FUNCTION "PR_GestioSalvastampi_WW" : VOID
TITLE =Gestione Salvastampi Cliente*
AUTHOR : 'A.A.E'
FAMILY : SALVASTA
NAME : SALVASTA
VERSION : 0.1


VAR_TEMP
  ST_CTRL : BOOL ;	//START CONTROLLO
  Camma_PMS : BOOL ;	//Appoggio per camma a pms
  CTRL_Syncr : BOOL ;	//Controllo Sincronismo
  Ang_Fren : INT ;	//Angolo Frenatura a PMS
  CMD_Prg : BOOL ;	//Comando Programmazione Camma
  Antic_Dyn : INT ;	//Gradi Anticipo Camme Dinamiche
  Page_Ok : BOOL ;	//Pagina Visualizzata HMI Corretta
  Results : INT ;
  ByPass_Cntr : BOOL ;
END_VAR
BEGIN
NETWORK
TITLE =R/Reset allarmi salvastampo*
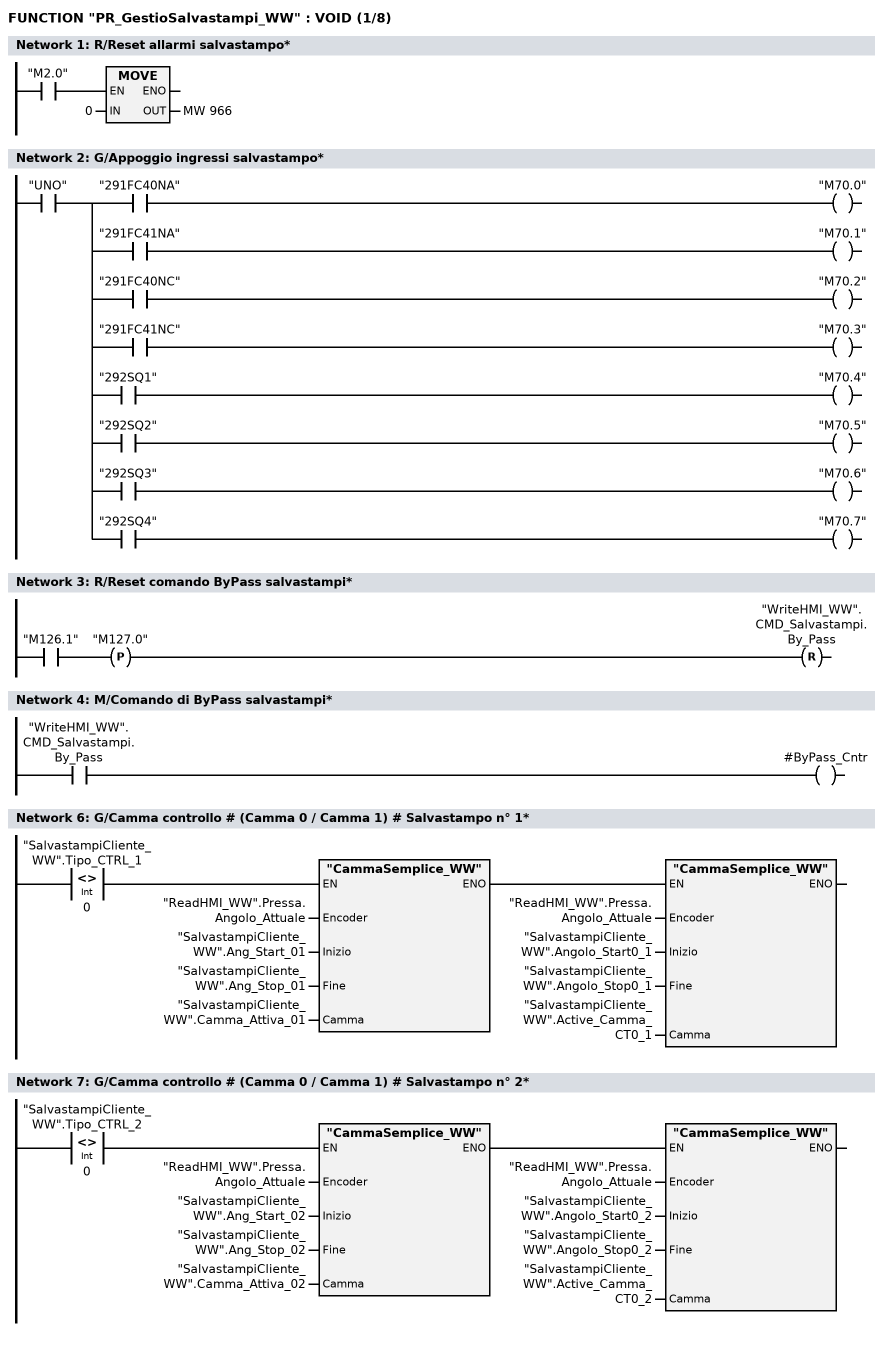
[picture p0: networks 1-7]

      U     "M2.0";
      SPBNB _001;
      L     0;
      T     MW   966;
_001: NOP   0;
NETWORK
TITLE =G/Appoggio ingressi salvastampo*

      U     "UNO";
      =     L     13.0;
      U     L     13.0;
      U     "291FC40NA";
      =     "M70.0";
      U     L     13.0;
      U     "291FC41NA";
      =     "M70.1";
      U     L     13.0;
      U     "291FC40NC";
      =     "M70.2";
      U     L     13.0;
      U     "291FC41NC";
      =     "M70.3";
      U     L     13.0;
      U     "292SQ1";
      =     "M70.4";
      U     L     13.0;
      U     "292SQ2";
      =     "M70.5";
      U     L     13.0;
      U     "292SQ3";
      =     "M70.6";
      U     L     13.0;
      U     "292SQ4";
      =     "M70.7";
NETWORK
TITLE =R/Reset comando ByPass salvastampi*

      U     "M126.1";
      FP    "M127.0";
      R     "WriteHMI_WW".CMD_Salvastampi.By_Pass;
NETWORK
TITLE =M/Comando di ByPass salvastampi*

      U     "WriteHMI_WW".CMD_Salvastampi.By_Pass;
      =     #ByPass_Cntr;
NETWORK
TITLE =######################## CAMME SALVASTAMPO #####################



NETWORK
TITLE =G/Camma controllo # (Camma 0 / Camma 1) # Salvastampo n° 1*

      U(    ;
      U(    ;
      L     "SalvastampiCliente_WW".Tipo_CTRL_1;
      L     0;
      <>I   ;
      )     ;
      SPBNB _002;
      CALL "CammaSemplice_WW" (
           Encoder                  := "ReadHMI_WW".Pressa.Angolo_Attuale,
           Inizio                   := "SalvastampiCliente_WW".Ang_Start_01,
           Fine                     := "SalvastampiCliente_WW".Ang_Stop_01,
           Camma                    := "SalvastampiCliente_WW".Camma_Attiva_01);
_002: U     BIE;
      )     ;
      SPBNB _003;
      CALL "CammaSemplice_WW" (
           Encoder                  := "ReadHMI_WW".Pressa.Angolo_Attuale,
           Inizio                   := "SalvastampiCliente_WW".Angolo_Start0_1,
           Fine                     := "SalvastampiCliente_WW".Angolo_Stop0_1,
           Camma                    := "SalvastampiCliente_WW".Active_Camma_CT0_1);
_003: NOP   0;
NETWORK
TITLE =G/Camma controllo # (Camma 0 / Camma 1) # Salvastampo n° 2*

      U(    ;
      U(    ;
      L     "SalvastampiCliente_WW".Tipo_CTRL_2;
      L     0;
      <>I   ;
      )     ;
      SPBNB _004;
      CALL "CammaSemplice_WW" (
           Encoder                  := "ReadHMI_WW".Pressa.Angolo_Attuale,
           Inizio                   := "SalvastampiCliente_WW".Ang_Start_02,
           Fine                     := "SalvastampiCliente_WW".Ang_Stop_02,
           Camma                    := "SalvastampiCliente_WW".Camma_Attiva_02);
_004: U     BIE;
      )     ;
      SPBNB _005;
      CALL "CammaSemplice_WW" (
           Encoder                  := "ReadHMI_WW".Pressa.Angolo_Attuale,
           Inizio                   := "SalvastampiCliente_WW".Angolo_Start0_2,
           Fine                     := "SalvastampiCliente_WW".Angolo_Stop0_2,
           Camma                    := "SalvastampiCliente_WW".Active_Camma_CT0_2);
_005: NOP   0;
NETWORK
TITLE =G/Camma controllo # (Camma 0 / Camma 1) # Salvastampo n° 3*
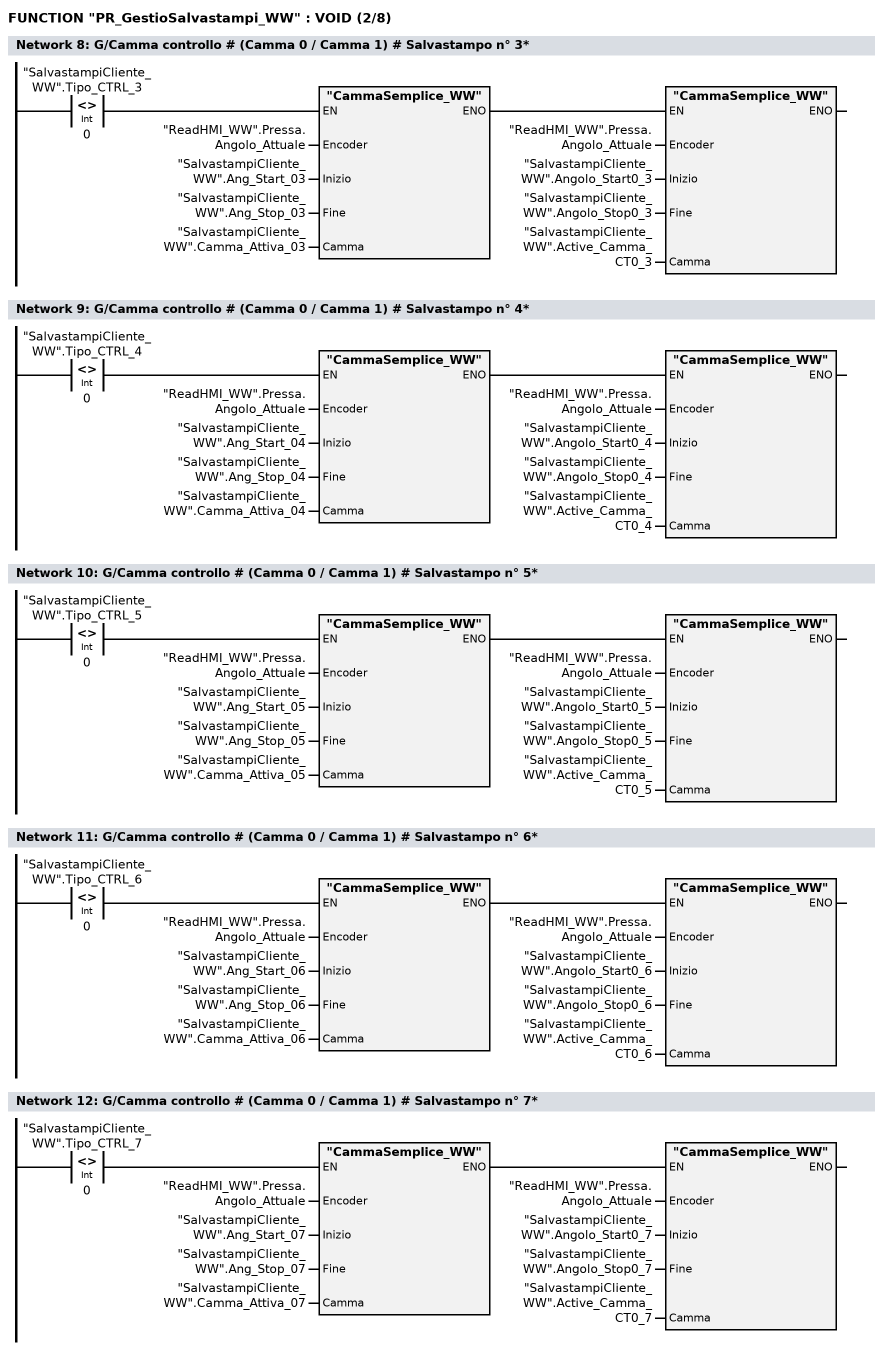
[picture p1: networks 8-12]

      U(    ;
      U(    ;
      L     "SalvastampiCliente_WW".Tipo_CTRL_3;
      L     0;
      <>I   ;
      )     ;
      SPBNB _006;
      CALL "CammaSemplice_WW" (
           Encoder                  := "ReadHMI_WW".Pressa.Angolo_Attuale,
           Inizio                   := "SalvastampiCliente_WW".Ang_Start_03,
           Fine                     := "SalvastampiCliente_WW".Ang_Stop_03,
           Camma                    := "SalvastampiCliente_WW".Camma_Attiva_03);
_006: U     BIE;
      )     ;
      SPBNB _007;
      CALL "CammaSemplice_WW" (
           Encoder                  := "ReadHMI_WW".Pressa.Angolo_Attuale,
           Inizio                   := "SalvastampiCliente_WW".Angolo_Start0_3,
           Fine                     := "SalvastampiCliente_WW".Angolo_Stop0_3,
           Camma                    := "SalvastampiCliente_WW".Active_Camma_CT0_3);
_007: NOP   0;
NETWORK
TITLE =G/Camma controllo # (Camma 0 / Camma 1) # Salvastampo n° 4*

      U(    ;
      U(    ;
      L     "SalvastampiCliente_WW".Tipo_CTRL_4;
      L     0;
      <>I   ;
      )     ;
      SPBNB _008;
      CALL "CammaSemplice_WW" (
           Encoder                  := "ReadHMI_WW".Pressa.Angolo_Attuale,
           Inizio                   := "SalvastampiCliente_WW".Ang_Start_04,
           Fine                     := "SalvastampiCliente_WW".Ang_Stop_04,
           Camma                    := "SalvastampiCliente_WW".Camma_Attiva_04);
_008: U     BIE;
      )     ;
      SPBNB _009;
      CALL "CammaSemplice_WW" (
           Encoder                  := "ReadHMI_WW".Pressa.Angolo_Attuale,
           Inizio                   := "SalvastampiCliente_WW".Angolo_Start0_4,
           Fine                     := "SalvastampiCliente_WW".Angolo_Stop0_4,
           Camma                    := "SalvastampiCliente_WW".Active_Camma_CT0_4);
_009: NOP   0;
NETWORK
TITLE =G/Camma controllo # (Camma 0 / Camma 1) # Salvastampo n° 5*

      U(    ;
      U(    ;
      L     "SalvastampiCliente_WW".Tipo_CTRL_5;
      L     0;
      <>I   ;
      )     ;
      SPBNB _00a;
      CALL "CammaSemplice_WW" (
           Encoder                  := "ReadHMI_WW".Pressa.Angolo_Attuale,
           Inizio                   := "SalvastampiCliente_WW".Ang_Start_05,
           Fine                     := "SalvastampiCliente_WW".Ang_Stop_05,
           Camma                    := "SalvastampiCliente_WW".Camma_Attiva_05);
_00a: U     BIE;
      )     ;
      SPBNB _00b;
      CALL "CammaSemplice_WW" (
           Encoder                  := "ReadHMI_WW".Pressa.Angolo_Attuale,
           Inizio                   := "SalvastampiCliente_WW".Angolo_Start0_5,
           Fine                     := "SalvastampiCliente_WW".Angolo_Stop0_5,
           Camma                    := "SalvastampiCliente_WW".Active_Camma_CT0_5);
_00b: NOP   0;
NETWORK
TITLE =G/Camma controllo # (Camma 0 / Camma 1) # Salvastampo n° 6*

      U(    ;
      U(    ;
      L     "SalvastampiCliente_WW".Tipo_CTRL_6;
      L     0;
      <>I   ;
      )     ;
      SPBNB _00c;
      CALL "CammaSemplice_WW" (
           Encoder                  := "ReadHMI_WW".Pressa.Angolo_Attuale,
           Inizio                   := "SalvastampiCliente_WW".Ang_Start_06,
           Fine                     := "SalvastampiCliente_WW".Ang_Stop_06,
           Camma                    := "SalvastampiCliente_WW".Camma_Attiva_06);
_00c: U     BIE;
      )     ;
      SPBNB _00d;
      CALL "CammaSemplice_WW" (
           Encoder                  := "ReadHMI_WW".Pressa.Angolo_Attuale,
           Inizio                   := "SalvastampiCliente_WW".Angolo_Start0_6,
           Fine                     := "SalvastampiCliente_WW".Angolo_Stop0_6,
           Camma                    := "SalvastampiCliente_WW".Active_Camma_CT0_6);
_00d: NOP   0;
NETWORK
TITLE =G/Camma controllo # (Camma 0 / Camma 1) # Salvastampo n° 7*

      U(    ;
      U(    ;
      L     "SalvastampiCliente_WW".Tipo_CTRL_7;
      L     0;
      <>I   ;
      )     ;
      SPBNB _00e;
      CALL "CammaSemplice_WW" (
           Encoder                  := "ReadHMI_WW".Pressa.Angolo_Attuale,
           Inizio                   := "SalvastampiCliente_WW".Ang_Start_07,
           Fine                     := "SalvastampiCliente_WW".Ang_Stop_07,
           Camma                    := "SalvastampiCliente_WW".Camma_Attiva_07);
_00e: U     BIE;
      )     ;
      SPBNB _00f;
      CALL "CammaSemplice_WW" (
           Encoder                  := "ReadHMI_WW".Pressa.Angolo_Attuale,
           Inizio                   := "SalvastampiCliente_WW".Angolo_Start0_7,
           Fine                     := "SalvastampiCliente_WW".Angolo_Stop0_7,
           Camma                    := "SalvastampiCliente_WW".Active_Camma_CT0_7);
_00f: NOP   0;
NETWORK
TITLE =G/Camma controllo # (Camma 0 / Camma 1) # Salvastampo n° 8*
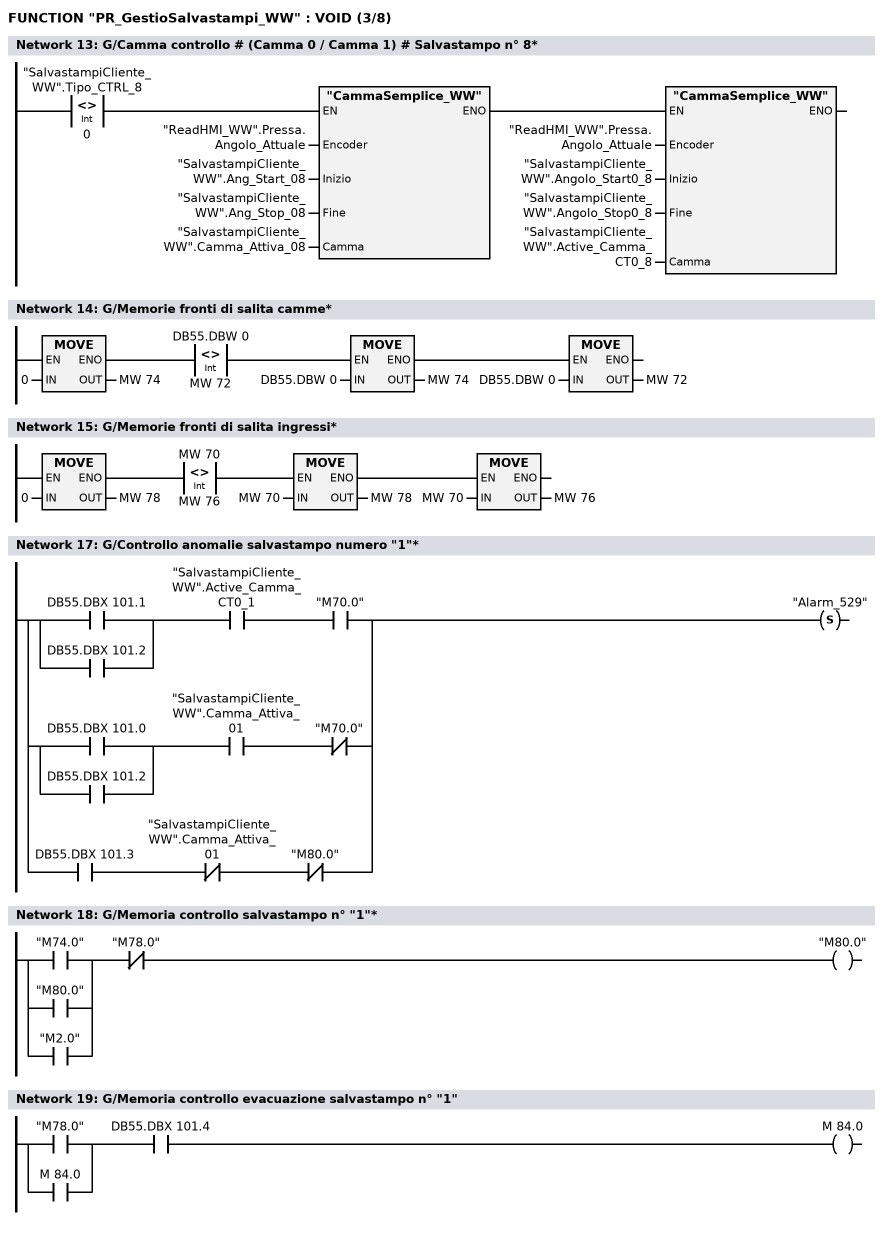
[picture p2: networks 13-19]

      U(    ;
      U(    ;
      L     "SalvastampiCliente_WW".Tipo_CTRL_8;
      L     0;
      <>I   ;
      )     ;
      SPBNB _010;
      CALL "CammaSemplice_WW" (
           Encoder                  := "ReadHMI_WW".Pressa.Angolo_Attuale,
           Inizio                   := "SalvastampiCliente_WW".Ang_Start_08,
           Fine                     := "SalvastampiCliente_WW".Ang_Stop_08,
           Camma                    := "SalvastampiCliente_WW".Camma_Attiva_08);
_010: U     BIE;
      )     ;
      SPBNB _011;
      CALL "CammaSemplice_WW" (
           Encoder                  := "ReadHMI_WW".Pressa.Angolo_Attuale,
           Inizio                   := "SalvastampiCliente_WW".Angolo_Start0_8,
           Fine                     := "SalvastampiCliente_WW".Angolo_Stop0_8,
           Camma                    := "SalvastampiCliente_WW".Active_Camma_CT0_8);
_011: NOP   0;
NETWORK
TITLE =G/Memorie fronti di salita camme*

      U(    ;
      U(    ;
      L     0;
      T     MW    74;
      SET   ;
      SAVE  ;
      CLR   ;
      U     BIE;
      )     ;
      U(    ;
      L     DB55.DBW    0;
      L     MW    72;
      <>I   ;
      )     ;
      SPBNB _012;
      L     DB55.DBW    0;
      T     MW    74;
      SET   ;
      SAVE  ;
      CLR   ;
_012: U     BIE;
      )     ;
      SPBNB _013;
      L     DB55.DBW    0;
      T     MW    72;
_013: NOP   0;
NETWORK
TITLE =G/Memorie fronti di salita ingressi*

      U(    ;
      U(    ;
      L     0;
      T     MW    78;
      SET   ;
      SAVE  ;
      CLR   ;
      U     BIE;
      )     ;
      U(    ;
      L     MW    70;
      L     MW    76;
      <>I   ;
      )     ;
      SPBNB _014;
      L     MW    70;
      T     MW    78;
      SET   ;
      SAVE  ;
      CLR   ;
_014: U     BIE;
      )     ;
      SPBNB _015;
      L     MW    70;
      T     MW    76;
_015: NOP   0;
NETWORK
TITLE =#################### CONTROLLO SALVASTAMPO #####################



NETWORK
TITLE =G/Controllo anomalie salvastampo numero "1"*

      U(    ;
      O     DB55.DBX  101.1;
      O     DB55.DBX  101.2;
      )     ;
      U     "SalvastampiCliente_WW".Active_Camma_CT0_1;
      U     "M70.0";
      O     ;
      U(    ;
      O     DB55.DBX  101.0;
      O     DB55.DBX  101.2;
      )     ;
      U     "SalvastampiCliente_WW".Camma_Attiva_01;
      UN    "M70.0";
      O     ;
      U     DB55.DBX  101.3;
      UN    "SalvastampiCliente_WW".Camma_Attiva_01;
      UN    "M80.0";
      S     "Alarm_529";
NETWORK
TITLE =G/Memoria controllo salvastampo n° "1"*

      U(    ;
      O     "M74.0";
      O     "M80.0";
      O     "M2.0";
      )     ;
      UN    "M78.0";
      =     "M80.0";
NETWORK
TITLE =G/Memoria controllo evacuazione salvastampo n° "1"

      U(    ;
      O     "M78.0";
      O     M     84.0;
      )     ;
      U     DB55.DBX  101.4;
      =     M     84.0;
NETWORK
TITLE =G/Controllo anomalie salvastampo numero "2"*
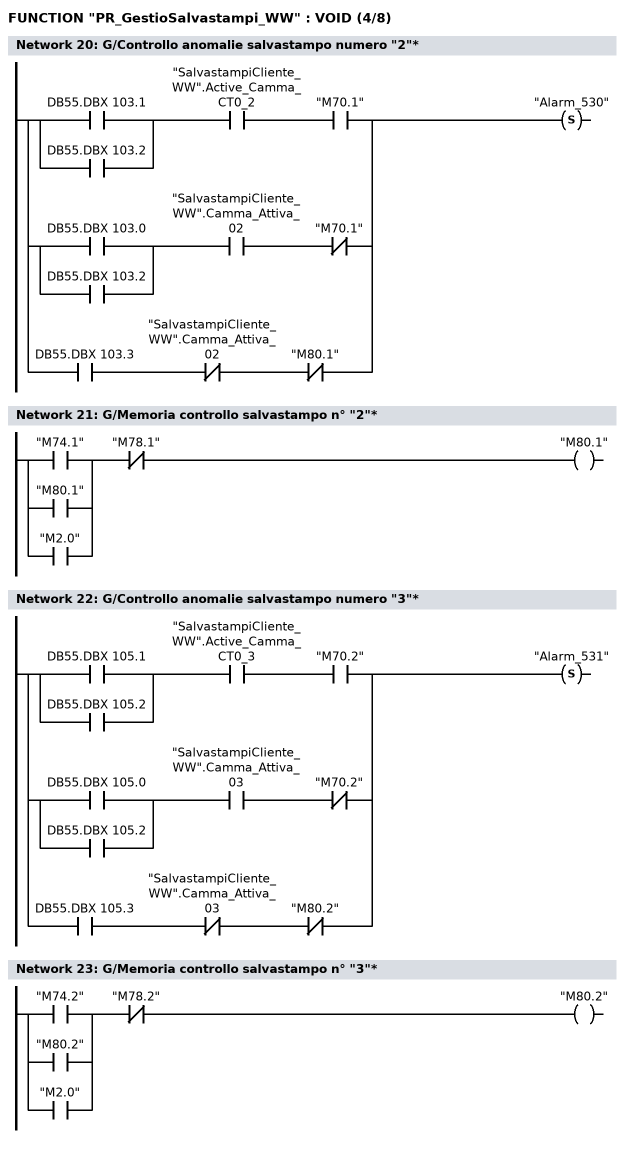
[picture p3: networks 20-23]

      U(    ;
      O     DB55.DBX  103.1;
      O     DB55.DBX  103.2;
      )     ;
      U     "SalvastampiCliente_WW".Active_Camma_CT0_2;
      U     "M70.1";
      O     ;
      U(    ;
      O     DB55.DBX  103.0;
      O     DB55.DBX  103.2;
      )     ;
      U     "SalvastampiCliente_WW".Camma_Attiva_02;
      UN    "M70.1";
      O     ;
      U     DB55.DBX  103.3;
      UN    "SalvastampiCliente_WW".Camma_Attiva_02;
      UN    "M80.1";
      S     "Alarm_530";
NETWORK
TITLE =G/Memoria controllo salvastampo n° "2"*

      U(    ;
      O     "M74.1";
      O     "M80.1";
      O     "M2.0";
      )     ;
      UN    "M78.1";
      =     "M80.1";
NETWORK
TITLE =G/Controllo anomalie salvastampo numero "3"*

      U(    ;
      O     DB55.DBX  105.1;
      O     DB55.DBX  105.2;
      )     ;
      U     "SalvastampiCliente_WW".Active_Camma_CT0_3;
      U     "M70.2";
      O     ;
      U(    ;
      O     DB55.DBX  105.0;
      O     DB55.DBX  105.2;
      )     ;
      U     "SalvastampiCliente_WW".Camma_Attiva_03;
      UN    "M70.2";
      O     ;
      U     DB55.DBX  105.3;
      UN    "SalvastampiCliente_WW".Camma_Attiva_03;
      UN    "M80.2";
      S     "Alarm_531";
NETWORK
TITLE =G/Memoria controllo salvastampo n° "3"*

      U(    ;
      O     "M74.2";
      O     "M80.2";
      O     "M2.0";
      )     ;
      UN    "M78.2";
      =     "M80.2";
NETWORK
TITLE =G/Controllo anomalie salvastampo numero "4"*
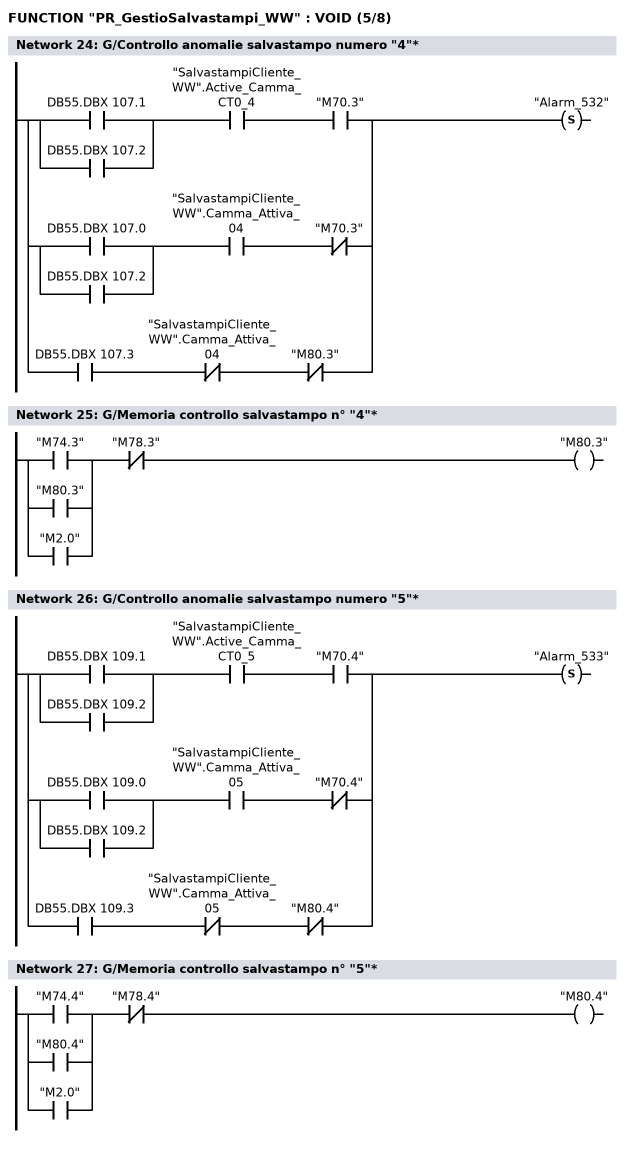
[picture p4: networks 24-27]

      U(    ;
      O     DB55.DBX  107.1;
      O     DB55.DBX  107.2;
      )     ;
      U     "SalvastampiCliente_WW".Active_Camma_CT0_4;
      U     "M70.3";
      O     ;
      U(    ;
      O     DB55.DBX  107.0;
      O     DB55.DBX  107.2;
      )     ;
      U     "SalvastampiCliente_WW".Camma_Attiva_04;
      UN    "M70.3";
      O     ;
      U     DB55.DBX  107.3;
      UN    "SalvastampiCliente_WW".Camma_Attiva_04;
      UN    "M80.3";
      S     "Alarm_532";
NETWORK
TITLE =G/Memoria controllo salvastampo n° "4"*

      U(    ;
      O     "M74.3";
      O     "M80.3";
      O     "M2.0";
      )     ;
      UN    "M78.3";
      =     "M80.3";
NETWORK
TITLE =G/Controllo anomalie salvastampo numero "5"*

      U(    ;
      O     DB55.DBX  109.1;
      O     DB55.DBX  109.2;
      )     ;
      U     "SalvastampiCliente_WW".Active_Camma_CT0_5;
      U     "M70.4";
      O     ;
      U(    ;
      O     DB55.DBX  109.0;
      O     DB55.DBX  109.2;
      )     ;
      U     "SalvastampiCliente_WW".Camma_Attiva_05;
      UN    "M70.4";
      O     ;
      U     DB55.DBX  109.3;
      UN    "SalvastampiCliente_WW".Camma_Attiva_05;
      UN    "M80.4";
      S     "Alarm_533";
NETWORK
TITLE =G/Memoria controllo salvastampo n° "5"*

      U(    ;
      O     "M74.4";
      O     "M80.4";
      O     "M2.0";
      )     ;
      UN    "M78.4";
      =     "M80.4";
NETWORK
TITLE =G/Controllo anomalie salvastampo numero "6"*
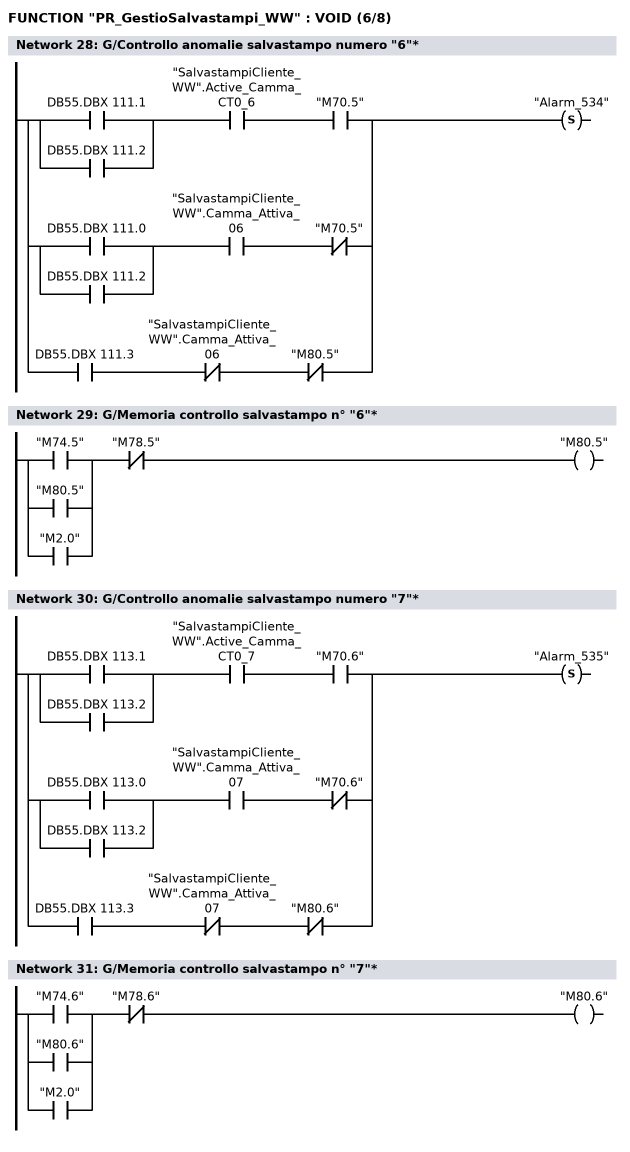
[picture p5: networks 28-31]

      U(    ;
      O     DB55.DBX  111.1;
      O     DB55.DBX  111.2;
      )     ;
      U     "SalvastampiCliente_WW".Active_Camma_CT0_6;
      U     "M70.5";
      O     ;
      U(    ;
      O     DB55.DBX  111.0;
      O     DB55.DBX  111.2;
      )     ;
      U     "SalvastampiCliente_WW".Camma_Attiva_06;
      UN    "M70.5";
      O     ;
      U     DB55.DBX  111.3;
      UN    "SalvastampiCliente_WW".Camma_Attiva_06;
      UN    "M80.5";
      S     "Alarm_534";
NETWORK
TITLE =G/Memoria controllo salvastampo n° "6"*

      U(    ;
      O     "M74.5";
      O     "M80.5";
      O     "M2.0";
      )     ;
      UN    "M78.5";
      =     "M80.5";
NETWORK
TITLE =G/Controllo anomalie salvastampo numero "7"*

      U(    ;
      O     DB55.DBX  113.1;
      O     DB55.DBX  113.2;
      )     ;
      U     "SalvastampiCliente_WW".Active_Camma_CT0_7;
      U     "M70.6";
      O     ;
      U(    ;
      O     DB55.DBX  113.0;
      O     DB55.DBX  113.2;
      )     ;
      U     "SalvastampiCliente_WW".Camma_Attiva_07;
      UN    "M70.6";
      O     ;
      U     DB55.DBX  113.3;
      UN    "SalvastampiCliente_WW".Camma_Attiva_07;
      UN    "M80.6";
      S     "Alarm_535";
NETWORK
TITLE =G/Memoria controllo salvastampo n° "7"*

      U(    ;
      O     "M74.6";
      O     "M80.6";
      O     "M2.0";
      )     ;
      UN    "M78.6";
      =     "M80.6";
NETWORK
TITLE =G/Controllo anomalie salvastampo numero "8"*
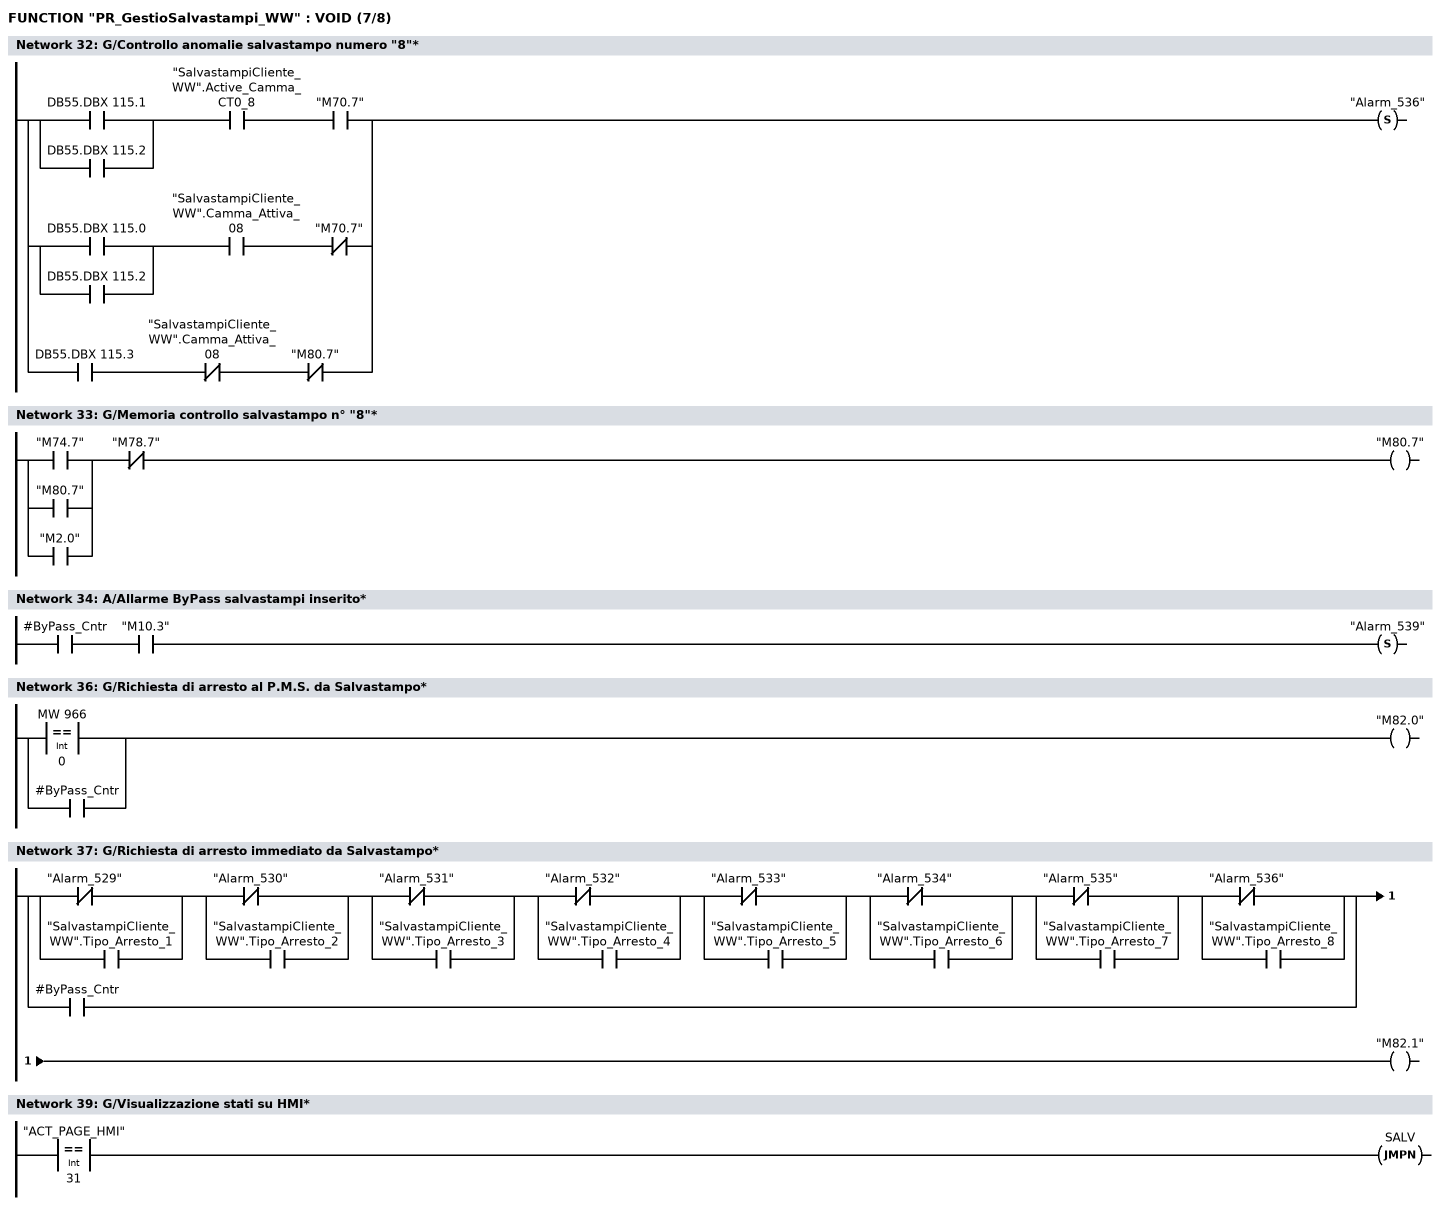
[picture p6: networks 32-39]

      U(    ;
      O     DB55.DBX  115.1;
      O     DB55.DBX  115.2;
      )     ;
      U     "SalvastampiCliente_WW".Active_Camma_CT0_8;
      U     "M70.7";
      O     ;
      U(    ;
      O     DB55.DBX  115.0;
      O     DB55.DBX  115.2;
      )     ;
      U     "SalvastampiCliente_WW".Camma_Attiva_08;
      UN    "M70.7";
      O     ;
      U     DB55.DBX  115.3;
      UN    "SalvastampiCliente_WW".Camma_Attiva_08;
      UN    "M80.7";
      S     "Alarm_536";
NETWORK
TITLE =G/Memoria controllo salvastampo n° "8"*

      U(    ;
      O     "M74.7";
      O     "M80.7";
      O     "M2.0";
      )     ;
      UN    "M78.7";
      =     "M80.7";
NETWORK
TITLE =A/Allarme ByPass salvastampi inserito*

      U     #ByPass_Cntr;
      U     "M10.3";
      S     "Alarm_539";
NETWORK
TITLE =###################### CONSENSI SALVASTAMPO ####################



NETWORK
TITLE =G/Richiesta di arresto al P.M.S. da Salvastampo*

      O(    ;
      L     MW   966;
      L     0;
      ==I   ;
      )     ;
      O     #ByPass_Cntr;
      =     "M82.0";
NETWORK
TITLE =G/Richiesta di arresto immediato da Salvastampo*

      U(    ;
      ON    "Alarm_529";
      O     "SalvastampiCliente_WW".Tipo_Arresto_1;
      )     ;
      U(    ;
      ON    "Alarm_530";
      O     "SalvastampiCliente_WW".Tipo_Arresto_2;
      )     ;
      U(    ;
      ON    "Alarm_531";
      O     "SalvastampiCliente_WW".Tipo_Arresto_3;
      )     ;
      U(    ;
      ON    "Alarm_532";
      O     "SalvastampiCliente_WW".Tipo_Arresto_4;
      )     ;
      U(    ;
      ON    "Alarm_533";
      O     "SalvastampiCliente_WW".Tipo_Arresto_5;
      )     ;
      U(    ;
      ON    "Alarm_534";
      O     "SalvastampiCliente_WW".Tipo_Arresto_6;
      )     ;
      U(    ;
      ON    "Alarm_535";
      O     "SalvastampiCliente_WW".Tipo_Arresto_7;
      )     ;
      U(    ;
      ON    "Alarm_536";
      O     "SalvastampiCliente_WW".Tipo_Arresto_8;
      )     ;
      O     #ByPass_Cntr;
      =     "M82.1";
NETWORK
TITLE =###################### VISUALIZZAZIONI HMI #####################



NETWORK
TITLE =G/Visualizzazione stati su HMI*

      L     "ACT_PAGE_HMI";
      L     31;
      ==I   ;
      SPBN  SALV;
NETWORK
TITLE =V/Stati monitor - Byte 001 - LED 024/031
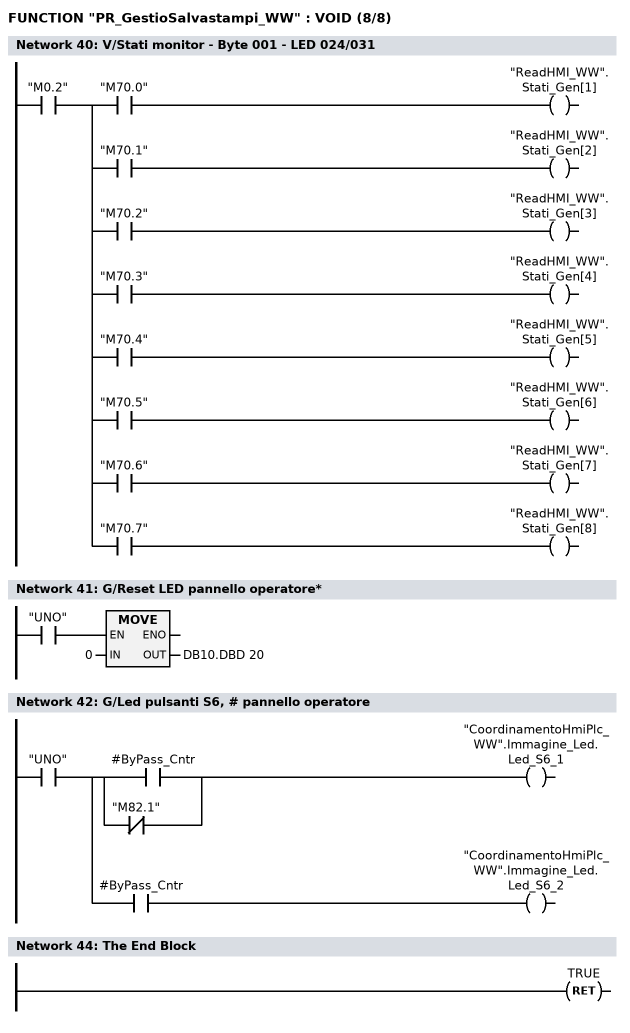
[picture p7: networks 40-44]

      U     "M0.2";
      =     L     13.0;
      U     L     13.0;
      U     "M70.0";
      =     "ReadHMI_WW".Stati_Gen[1];
      U     L     13.0;
      U     "M70.1";
      =     "ReadHMI_WW".Stati_Gen[2];
      U     L     13.0;
      U     "M70.2";
      =     "ReadHMI_WW".Stati_Gen[3];
      U     L     13.0;
      U     "M70.3";
      =     "ReadHMI_WW".Stati_Gen[4];
      U     L     13.0;
      U     "M70.4";
      =     "ReadHMI_WW".Stati_Gen[5];
      U     L     13.0;
      U     "M70.5";
      =     "ReadHMI_WW".Stati_Gen[6];
      U     L     13.0;
      U     "M70.6";
      =     "ReadHMI_WW".Stati_Gen[7];
      U     L     13.0;
      U     "M70.7";
      =     "ReadHMI_WW".Stati_Gen[8];
NETWORK
TITLE =G/Reset LED pannello operatore*

      U     "UNO";
      SPBNB _016;
      L     0;
      T     DB10.DBD   20;
_016: NOP   0;
NETWORK
TITLE =G/Led pulsanti S6, # pannello operatore

      U     "UNO";
      =     L     13.0;
      U     L     13.0;
      U(    ;
      O     #ByPass_Cntr;
      ON    "M82.1";
      )     ;
      =     "CoordinamentoHmiPlc_WW".Immagine_Led.Led_S6_1;
      U     L     13.0;
      U     #ByPass_Cntr;
      =     "CoordinamentoHmiPlc_WW".Immagine_Led.Led_S6_2;
NETWORK
TITLE =G/Fine salto animazioni HMI*

SALV: NOP   0;

NETWORK
TITLE =The End Block

      BEA   ;

END_FUNCTION

